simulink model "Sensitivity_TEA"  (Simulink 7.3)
settings: Solver=ode113  StartTime=0.0  StopTime=100000  RelTol=1e-3
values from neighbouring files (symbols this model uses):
  Ave = [    [vehicle_flex34.m]    (also in vehicle_rigid.m)
  Bve = [    [vehicle_flex34.m]    (also in vehicle_rigid.m)
  CB2L = [cpsi, -cphi*spsi,  sphi*spsi;          0,    cphi,      -sphi;          0,    sphi*cpsi,  cphi*cpsi]/cpsi    [Rigbod_Dynam_LVLH.m]    (also in start.m = eye(3); start2.m = eye(3); start3.m = eye(3); start1.m = eye(3))
  Cve = [    [vehicle_flex34.m]    (also in vehicle_rigid.m)
  Dve = [    [vehicle_flex34.m]    (also in vehicle_rigid.m)
  ini = [wbo; atto; Hco]    [start.m]    (also in start2.m; start3.m; start1.m)
  Kpqr = lqr(sys,Q0,R0)    [des.m]
  nt = 12    [start.m]    (also in start2.m; start3.m; start1.m)
  wo = 0.0011    [start.m]    (also in start2.m; start3.m; start1.m)
undefined symbols (not defined in the file or in its folder): Rigbod_Dynam_LVLH

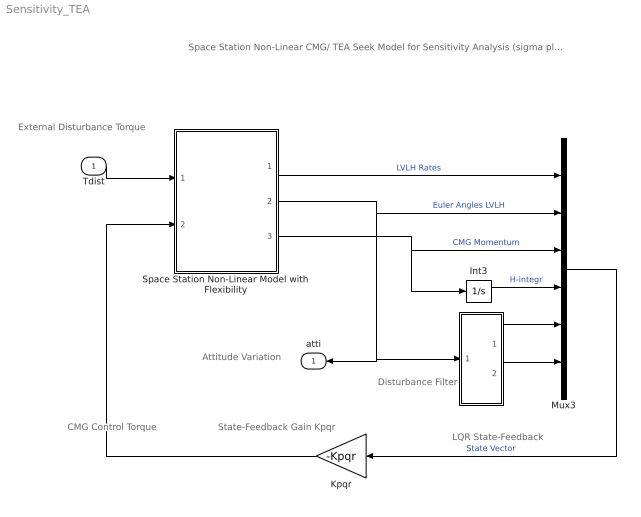
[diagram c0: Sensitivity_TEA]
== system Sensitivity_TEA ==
  note: Space Station Non-Linear CMG/ TEA Seek Model for Sensitivity Analysis (sigma plots)
  note: LQR State-Feedback
  note: CMG Control Torque
  note: Disturbance Filter
  note: External Disturbance Torque
  note: Attitude Variation
  note: State-Feedback Gain Kpqr
  Tdist : Inport  PortDimensions=3  OutDataType=sfix(16)  OutScaling=2^0
  " " : Subsystem
  Int3 : Integrator
  Kpqr : Gain  Gain=-Kpqr  Multiplication=Matrix(K*u)  ParameterDataType=sfix(16)  ParameterScaling=2^0  OutDataType=sfix(16)  OutScaling=2^0
  Mux3 : Mux  Inputs=[3, 3, 3, 3, 1, 1]
  Space Station Non-Linear Model with Flexibility : Subsystem
  atti : Outport  OutDataType=sfix(16)  OutScaling=2^0
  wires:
  Int3/1 -> Mux3/4  "H-integr"
  Space Station Non-Linear Model with Flexibility/3(Hcmg) -> Int3/1, Mux3/3  "CMG Momentum"
  Space Station Non-Linear Model with Flexibility/2(atti) -> Mux3/2, " "/1(the), atti/1  "Euler Angles LVLH"
  Kpqr/1 -> Space Station Non-Linear Model with Flexibility/2(Tcmg)
  Mux3/1 -> Kpqr/1  "State Vector"
  " "/1(a1) -> Mux3/5
  " "/2(a2) -> Mux3/6
  Space Station Non-Linear Model with Flexibility/1(wlv) -> Mux3/1  "LVLH Rates"
  Tdist/1 -> Space Station Non-Linear Model with Flexibility/1(Tdist)

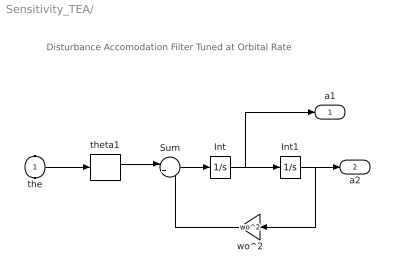
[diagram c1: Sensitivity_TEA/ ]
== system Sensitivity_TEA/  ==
  note: Disturbance Accomodation Filter Tuned at Orbital Rate
  the : Inport  OutDataType=sfix(16)  OutScaling=2^0
  Int : Integrator
  Int1 : Integrator
  Sum : Sum  Inputs=|+-  OutDataType=sfix(16)  OutScaling=2^0
  theta1 : Selector  InputPortWidth=3  IndexOptions=Index vector (dialog)  Indices=[2]  OutputSizes=1
  wo^2 : Gain  Gain=wo^2  ParameterDataType=sfix(16)  ParameterScaling=2^0  OutDataType=sfix(16)  OutScaling=2^0
  a1 : Outport  OutDataType=sfix(16)  OutScaling=2^0
  a2 : Outport  Port=2  OutDataType=sfix(16)  OutScaling=2^0
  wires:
  Int/1 -> Int1/1, a1/1
  Sum/1 -> Int/1
  Int1/1 -> wo^2/1, a2/1
  wo^2/1 -> Sum/2
  theta1/1 -> Sum/1
  the/1 -> theta1/1

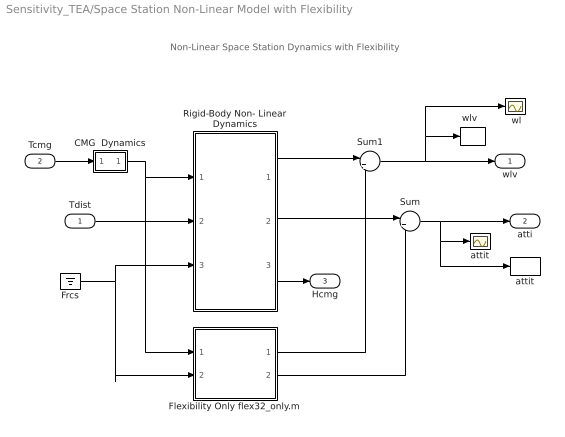
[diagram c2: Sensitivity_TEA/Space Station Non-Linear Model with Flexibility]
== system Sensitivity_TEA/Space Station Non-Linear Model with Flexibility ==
  note: Non-Linear Space Station Dynamics with Flexibility
  Tdist : Inport  OutDataType=sfix(16)  OutScaling=2^0
  Tcmg : Inport  Port=2  OutDataType=sfix(16)  OutScaling=2^0
  " attit " : Scope
  " wl" : Scope
  CMG  Dynamics : Subsystem
  Flexibility Only flex32_only.m : Subsystem
  Frcs : Ground
  Rigid-Body Non- Linear Dynamics : Subsystem
  Sum : Sum  Inputs=|++  OutDataType=sfix(16)  OutScaling=2^0
  Sum1 : Sum  Inputs=|++  OutDataType=sfix(16)  OutScaling=2^0
  attit : ToWorkspace  VariableName=theta  SampleTime=-1  SaveFormat=Array
  "wlv  " : ToWorkspace  VariableName=wl  SampleTime=-1  SaveFormat=Array
  wlv : Outport  OutDataType=sfix(16)  OutScaling=2^0
  atti : Outport  Port=2  OutDataType=sfix(16)  OutScaling=2^0
  Hcmg : Outport  Port=3  OutDataType=sfix(16)  OutScaling=2^0
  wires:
  Frcs/1 -> Rigid-Body Non- Linear Dynamics/3(Frcs), Flexibility Only flex32_only.m/2(Frcs)
  Rigid-Body Non- Linear Dynamics/2(atti-lv) -> Sum/1
  Flexibility Only flex32_only.m/2(att) -> Sum/2
  Sum/1 -> atti/1, " attit "/1, attit/1
  Sum1/1 -> wlv/1, "wlv  "/1, " wl"/1
  Tcmg/1 -> CMG  Dynamics/1(I)
  Rigid-Body Non- Linear Dynamics/1(w-lv) -> Sum1/1
  Flexibility Only flex32_only.m/1(wbf) -> Sum1/2
  Rigid-Body Non- Linear Dynamics/3(Hcmg) -> Hcmg/1
  CMG  Dynamics/1(O) -> Rigid-Body Non- Linear Dynamics/1(Tcmg), Flexibility Only flex32_only.m/1(Tcmg)
  Tdist/1 -> Rigid-Body Non- Linear Dynamics/2(Tdist)

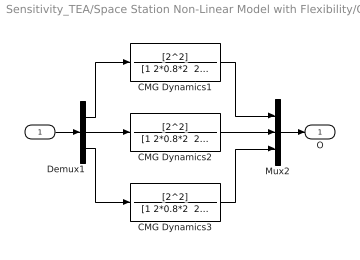
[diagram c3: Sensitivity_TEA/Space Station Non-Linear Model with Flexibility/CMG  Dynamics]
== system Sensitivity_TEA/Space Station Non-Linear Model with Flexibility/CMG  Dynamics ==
  I : Inport  OutDataType=sfix(16)  OutScaling=2^0
  CMG Dynamics1 : TransferFcn  Numerator=[2^2]  Denominator="[1 2*0.8*2  2^2]"
  CMG Dynamics2 : TransferFcn  Numerator=[2^2]  Denominator="[1 2*0.8*2  2^2]"
  CMG Dynamics3 : TransferFcn  Numerator=[2^2]  Denominator="[1 2*0.8*2  2^2]"
  Demux1 : Demux  Outputs=3
  Mux2 : Mux  Inputs=3
  O : Outport  OutDataType=sfix(16)  OutScaling=2^0
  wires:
  Mux2/1 -> O/1
  I/1 -> Demux1/1
  Demux1/3 -> CMG Dynamics3/1
  Demux1/1 -> CMG Dynamics1/1
  Demux1/2 -> CMG Dynamics2/1
  CMG Dynamics1/1 -> Mux2/1
  CMG Dynamics3/1 -> Mux2/3
  CMG Dynamics2/1 -> Mux2/2

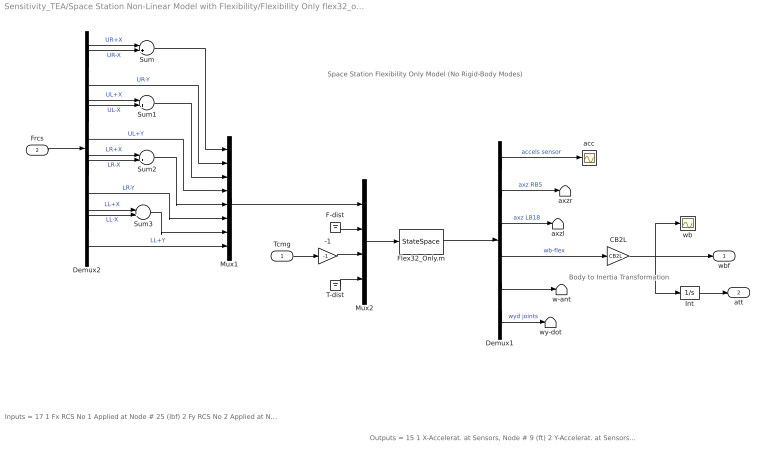
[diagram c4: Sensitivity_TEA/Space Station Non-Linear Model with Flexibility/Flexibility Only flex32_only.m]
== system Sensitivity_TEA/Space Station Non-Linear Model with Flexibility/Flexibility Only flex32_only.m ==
  note: Outputs = 15 1 X-Accelerat. at Sensors, Node # 9 (ft) 2 Y-Accelerat. at Sensors, Node # 9 (ft) 3 Z-Accelerat. at Sensors, Node # 9 (ft) 4 X-Accelerat. at Right Boom End, Node # 5 (ft) 5 Z-Accelerat. at Right Boom End, Node # 5 (ft) 6 X-Accelerat. at Left Boom End, Node # 18 (ft) 7 Z-Accelerat. at Left Boom End, Node # 18 (ft) 8 X-Rot. Rate at Sensors, Node # 9 (radian) 9 Y-Rot. Rate at Sensors, Node # 9 (radian) 10 Z-Rot. Rate at Sensors, Node # 9 (radian) 11 X-Rot. Rate at Antena Bot-Left, Node # 24 (radian) 12 Y-Rot. Rate at Antena Bot-Left, Node # 24 (radian) 13 Z-Rot. Rate at Antena Bot-Left, Node # 24 (radian) 14 Y-Rot.Accel. at Right Joint, Node # 7 (radian) 15 Y-Rot.Accel. at Left Joint, Node # 16 (radian)
  note: Inputs = 17 1 Fx RCS No 1 Applied at Node # 25 (lbf) 2 Fy RCS No 2 Applied at Node # 25 (lbf) 3 Fx RCS No 3 Applied at Node # 26 (lbf) 4 Fy RCS No 4 Applied at Node # 26 (lbf) 5 Fx RCS No 5 Applied at Node # 27 (lbf) 6 Fy RCS No 6 Applied at Node # 27 (lbf) 7 Fx RCS No 7 Applied at Node # 28 (lbf) 8 Fy RCS No 8 Applied at Node # 28 (lbf) 9 Fx Disturb. No 9 at Node # 21 (lbf) 10 Fy Disturb. No 10 at Node # 21 (lbf) 11 Fz Disturb. No 11 at Node # 21 (lbf) 12 Torq-x No 1 CMG Applied at Node # 10 (ft-lb) 13 Torq-y No 2 CMG Applied at Node # 10 (ft-lb) 14 Torq-z No 3 CMG Applied at Node # 10 (ft-lb) 15 Torq-x No 4 Gimbal Dist. at Node # 1 (ft-lb) 16 Torq-y No 5 Gimbal Dist. at Node # 1 (ft-lb) 17 Torq-z No 6 Gimbal Dist. at Node # 1 (ft-lb)
  note: Space Station Flexibility Only Model (No Rigid-Body Modes)
  note: Body to Inertia Transformation
  Tcmg : Inport  OutDataType=sfix(16)  OutScaling=2^0
  Frcs : Inport  Port=2  OutDataType=sfix(16)  OutScaling=2^0
  -1 : Gain  Gain=-1  ParameterDataType=sfix(16)  ParameterScaling=2^0  OutDataType=sfix(16)  OutScaling=2^0
  CB2L : Gain  Gain=CB2L  Multiplication=Matrix(K*u)  ParameterDataType=sfix(16)  ParameterScaling=2^0  OutDataType=sfix(16)  OutScaling=2^0
  Demux1 : Demux  Outputs=[3, 2, 2, 3, 3, 2]
  Demux2 : Demux  Outputs=12
  F-dist : Ground
  Flex32_Only.m : StateSpace  A=Ave  B=Bve  C=Cve  D=Dve
  Int : Integrator
  Mux1 : Mux  Inputs=8
  Mux2 : Mux  Inputs=[8, 3, 3, 3]
  Sum{,1..3} (4 alike) : Sum  Inputs=|+-  OutDataType=sfix(16)  OutScaling=2^0
  T-dist : Ground
  acc : Scope
  axzl : Terminator
  axzr : Terminator
  w-ant : Terminator
  wb : Scope
  wy-dot : Terminator
  wbf : Outport  OutDataType=sfix(16)  OutScaling=2^0
  att : Outport  Port=2  OutDataType=sfix(16)  OutScaling=2^0
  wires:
  Demux1/6 -> wy-dot/1  "wyd joints"
  Demux1/5 -> w-ant/1
  T-dist/1 -> Mux2/4
  F-dist/1 -> Mux2/2
  Demux1/3 -> axzl/1  "axz LB18"
  Demux1/2 -> axzr/1  "axz RB5"
  Tcmg/1 -> -1/1
  Demux1/4 -> CB2L/1  "wb-flex"
  Demux1/1 -> acc/1  "accels sensor"
  Flex32_Only.m/1 -> Demux1/1
  Mux2/1 -> Flex32_Only.m/1
  Mux1/1 -> Mux2/1
  Frcs/1 -> Demux2/1
  Demux2/6 -> Mux1/4  "UL+Y"
  Demux2/9 -> Mux1/6  "LR-Y"
  Demux2/12 -> Mux1/8  "LL+Y"
  Demux2/3 -> Mux1/2  "UR-Y"
  Demux2/1 -> Sum/1  "UR+X"
  Demux2/2 -> Sum/2  "UR-X"
  Sum/1 -> Mux1/1
  Demux2/4 -> Sum1/1  "UL+X"
  Demux2/5 -> Sum1/2  "UL-X"
  Sum1/1 -> Mux1/3
  Demux2/7 -> Sum2/1  "LR+X"
  Demux2/8 -> Sum2/2  "LR-X"
  Demux2/10 -> Sum3/1  "LL+X"
  Demux2/11 -> Sum3/2  "LL-X"
  Sum3/1 -> Mux1/7
  Sum2/1 -> Mux1/5
  Int/1 -> att/1
  -1/1 -> Mux2/3
  CB2L/1 -> wb/1, wbf/1, Int/1

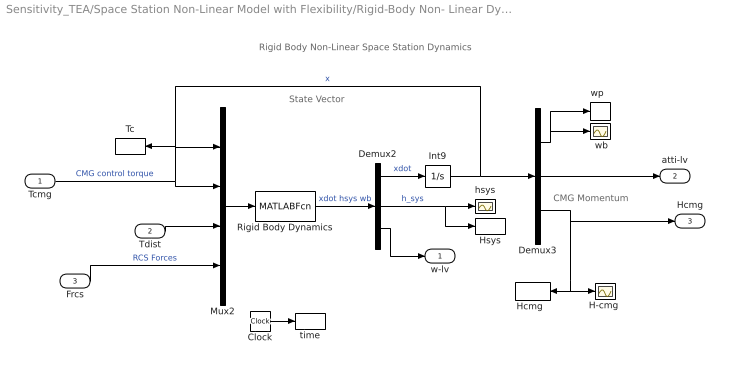
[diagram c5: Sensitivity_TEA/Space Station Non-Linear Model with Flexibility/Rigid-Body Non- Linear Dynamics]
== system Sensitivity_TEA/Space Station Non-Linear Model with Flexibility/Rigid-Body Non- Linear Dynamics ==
  note: CMG Momentum
  note: State Vector
  note: Rigid Body Non-Linear Space Station Dynamics
  Tcmg : Inport  PortDimensions=3  OutDataType=sfix(16)  OutScaling=2^0
  Tdist : Inport  Port=2  PortDimensions=3  OutDataType=sfix(16)  OutScaling=2^0
  Frcs : Inport  Port=3  PortDimensions=nt  OutDataType=sfix(16)  OutScaling=2^0
  " wb" : Scope
  Clock : Clock
  Demux2 : Demux  Outputs=[9,3,3]
  Demux3 : Demux  Outputs=[3,3,3]
  "H-cmg " : Scope
  "Hcmg  " : ToWorkspace  VariableName=Hcmg  SampleTime=-1  SaveFormat=Array
  Hsys : ToWorkspace  VariableName=Hsys  SampleTime=-1  SaveFormat=Array
  Int9 : Integrator  InitialCondition=ini
  Mux2 : Mux  Inputs=[9, 3, 3, nt]
  Rigid Body Dynamics : MATLABFcn  MATLABFcn=Rigbod_Dynam_LVLH( u(1:9), u(10:12), u(13:15), u(16:15+nt) )  OutputDimensions=15
  Tc : ToWorkspace  VariableName=Tcmg  SampleTime=-1  SaveFormat=Array
  hsys : Scope
  time : ToWorkspace  VariableName=time  SampleTime=-1  SaveFormat=Array
  "wp  " : ToWorkspace  VariableName=wb  SampleTime=-1  SaveFormat=Array
  w-lv : Outport  OutDataType=sfix(16)  OutScaling=2^0
  atti-lv : Outport  Port=2  OutDataType=sfix(16)  OutScaling=2^0
  Hcmg : Outport  Port=3  OutDataType=sfix(16)  OutScaling=2^0
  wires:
  Mux2/1 -> Rigid Body Dynamics/1
  Clock/1 -> time/1
  Frcs/1 -> Mux2/4  "RCS Forces"
  Demux3/3 -> Hcmg/1, "H-cmg "/1, "Hcmg  "/1
  Demux3/2 -> atti-lv/1
  Demux2/2 -> Hsys/1, hsys/1  "h_sys"
  Demux2/3 -> w-lv/1
  Tcmg/1 -> Mux2/2, Tc/1  "CMG control torque"
  Int9/1 -> Mux2/1, Demux3/1  "x"
  Demux2/1 -> Int9/1  "xdot"
  Rigid Body Dynamics/1 -> Demux2/1  "xdot hsys wb"
  Demux3/1 -> " wb"/1, "wp  "/1
  Tdist/1 -> Mux2/3
